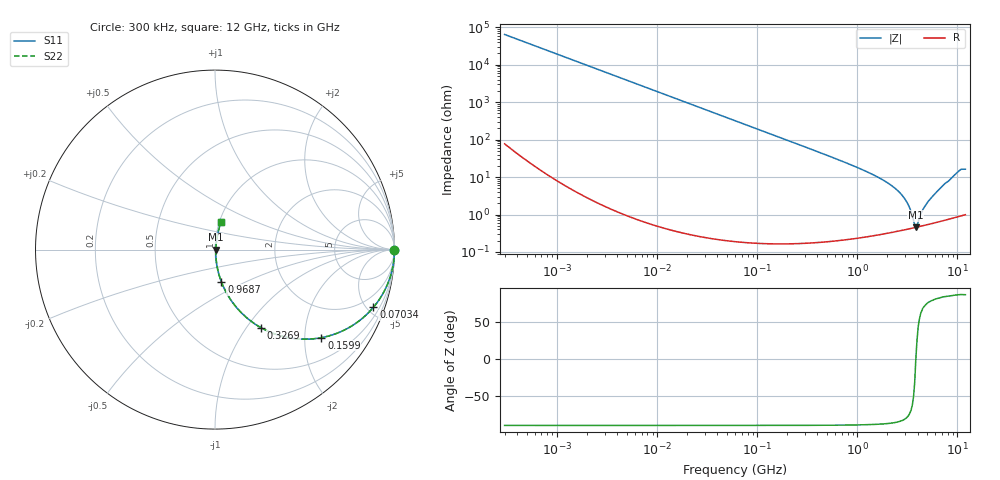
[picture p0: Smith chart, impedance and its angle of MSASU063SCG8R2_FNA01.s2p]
! MSASU063SCG8R2_FNA01  S-PARAMETER MODEL  ( Standard Model )
! Model Generated by TAIYO YUDEN Corporation (http://www.ty-top.com)
! Version 1.0
! TAIYO YUDEN Control No. 240819
! Copyright(c) 2024 TAIYO YUDEN CO.,LTD. All Rights Reserved.
! Product Description (link to TY-COMPAS)
! https://ds.yuden.co.jp/TYCOMPAS/or/detail?pn=MSASU063SCG8R2DFNA01&u=M
! Products Name : Multilayer Ceramic Capacitors
! Characteristics :
!  Capacitance : 8.2 [pF] , Rated Voltage : 50 [V] , TCC : CG / C0G
!  Case Size : 0.6 x 0.3 / 0.024 x 0.012 [mm/inch] , Thickness : 0.3 / 0.012 [mm/inch]
!  (Conditions: Temperature = 25 [degC] , DC Bias Voltage = 0 [V])
! External Node Assignments :
!  1  o---| |---o  2
! GND o---------o GND
! Frequency Range : 0.3MHz  -  12000MHz  [ 401 STEP ]
# MHZ S RI R 50
! Freq[MHz].  S11 Real  S11 Imag  S21 Real  S21 Imag  S12 Real  S12 Imag  S22 Real  S22 Imag
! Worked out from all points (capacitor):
!   401 points, 300 kHz to 12 GHz, reference 50 ohm
!   read as one part in series: C = 8.24 pF near 316.3 kHz
!   lowest |Z| = 453 mohm at 3.841 GHz (marker M1)
!   series resonance near 3.84 GHz, so ESL is about 210 pH
!   S11 on the Smith chart (normalised r, x): 300 kHz: open; 70.34 MHz: 1.00, -5.49; 159.9 MHz: 1.00, -2.41; 326.9 MHz: 1.00, -1.17; 968.7 MHz: 1.00, -0.37; 12 GHz: 1.02, +0.32
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0.3  1 -0.00155  4.27e-06 0.00155  4.27e-06 0.00155  1 -0.00155
1.769972  0.9999 -0.00916  8.67e-05 0.00916  8.67e-05 0.00916  0.9999 -0.00916
10.44266  0.9971 -0.0539  0.00293 0.0539  0.00293 0.0539  0.9971 -0.0539
27.10171  0.9807 -0.1376  0.0193 0.1376  0.0193 0.1376  0.9807 -0.1376
60  0.9119 -0.2832  0.0881 0.2832  0.0881 0.2832  0.9119 -0.2832
70.33673  0.8827 -0.3214  0.1173 0.3214  0.1173 0.3214  0.8827 -0.3214
159.8975  0.5925 -0.4907  0.4075 0.4907  0.4075 0.4907  0.5925 -0.4907
326.9496  0.2567 -0.4353  0.7433 0.4353  0.7433 0.4353  0.2567 -0.4353
353.9943  0.2272 -0.4174  0.7728 0.4174  0.7728 0.4174  0.2272 -0.4174
555.3718  0.1053 -0.3042  0.8947 0.3042  0.8947 0.3042  0.1053 -0.3042
968.706  0.0358 -0.1797  0.9642 0.1797  0.9642 0.1797  0.0358 -0.1797
2088.533  0.00741 -0.0645  0.9926 0.0645  0.9926 0.0645  0.00741 -0.0645
2581.562  0.00526 -0.0407  0.9947 0.0407  0.9947 0.0407  0.00526 -0.0407
3026.31  0.00451 -0.0241  0.9955 0.0241  0.9955 0.0241  0.00451 -0.0241
3364.605  0.00435 -0.0133  0.9956 0.0133  0.9956 0.0133  0.00435 -0.0133
3740.715  0.00445 -0.00273  0.9956 0.00273  0.9956 0.00273  0.00445 -0.00273
3841.137  0.00451 4.05e-05  0.9955 -4.05e-05  0.9955 -4.05e-05  0.00451 4.05e-05
4050.141  0.00468 0.00433  0.9953 -0.00433  0.9953 -0.00433  0.00468 0.00433
4747.894  0.0054 0.0158  0.9946 -0.0158  0.9946 -0.0158  0.0054 0.0158
5715.274  0.00676 0.0309  0.9932 -0.0309  0.9932 -0.0309  0.00676 0.0309
10236.47  0.0279 0.1368  0.9721 -0.1368  0.9721 -0.1368  0.0279 0.1368
12000  0.0345 0.1545  0.9655 -0.1545  0.9655 -0.1545  0.0345 0.1545
